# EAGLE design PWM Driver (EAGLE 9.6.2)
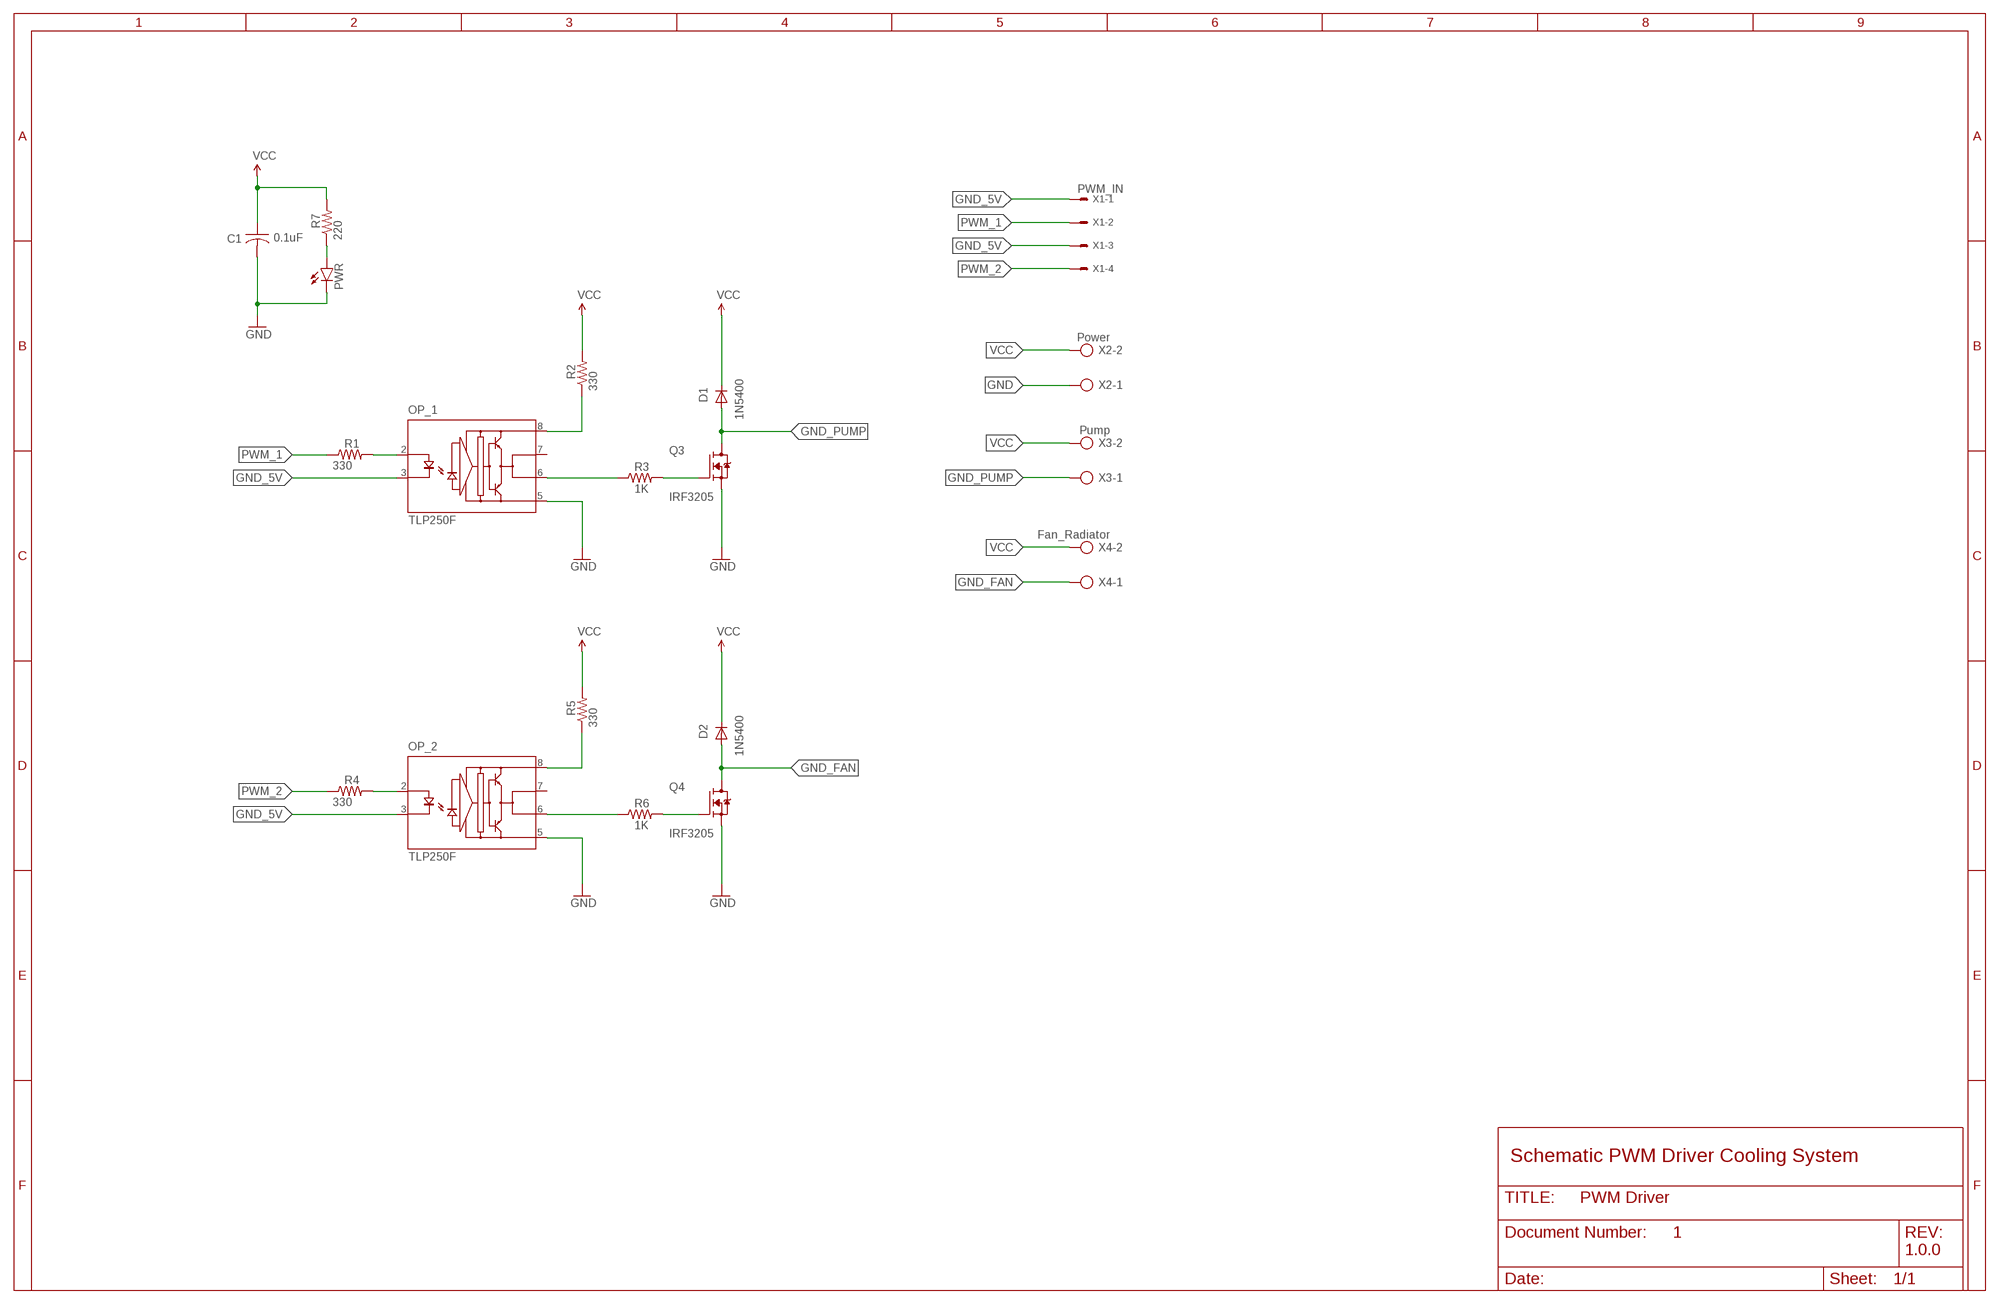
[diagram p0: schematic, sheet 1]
FRAME1 (FRAME_B_L): DESIGNER: PRATIK MAKWANA; DOC: 1; REV: 1.0.0

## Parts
C1  0.1uF  C-US050-030X075  [C050-030X075]
D1  1N5400  [DO201-15]
D2  1N5400  [DO201-15]
OP_1  TLP250F  [DIL08]
OP_2  TLP250F  [DIL08]
PWR  LED5MM  [LED5MM]
Q3  IRF3205  [TO254P1041X444X2933-3]
Q4  IRF3205  [TO254P1041X444X2933-3]
R1  330  R-US_0207/10  [0207/10]
R2  330  R-US_0411/15  [0411/15]
R3  1K  R-US_0411/15  [0411/15]
R4  330  R-US_0207/10  [0207/10]
R5  330  R-US_0411/15  [0411/15]
R6  1K  R-US_0411/15  [0411/15]
R7  220  R-US_0207/10  [0207/10]
X1  PWM_IN  22-23-2041  [22-23-2041]
X2  Power  AK500/2  [AK500/2]
X3  Pump  AK500/2  [AK500/2]
X4  Fan_Radiator  AK500/2  [AK500/2]

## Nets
GND: C1.2 OP_1.5(GND) OP_2.5(GND) PWR.K(C) Q3.3(S) Q4.3(S) X2.1
GND_5V: OP_1.3(K) OP_2.3(K) X1.1 X1.3
GND_FAN: D2.A Q4.2(D) X4.1
GND_PUMP: D1.A Q3.2(D) X3.1
N$1: OP_2.2(A) R4.2
N$2: OP_1.2(A) R1.2
N$3: OP_2.6(VO) R6.1
N$4: OP_1.6(VO) R3.1
N$5: Q3.1(G) R3.2
N$6: PWR.A R7.1
N$7: OP_1.8(VCC) R2.1
N$8: Q4.1(G) R6.2
N$9: OP_2.8(VCC) R5.1
PWM_1: R1.1 X1.2
PWM_2: R4.1 X1.4
VCC: C1.1 D1.C D2.C R2.2 R5.2 R7.2 X2.2 X3.2 X4.2
Unconnected: OP_1.7(VO') OP_2.7(VO')

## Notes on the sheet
- Schematic PWM Driver Cooling System

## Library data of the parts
C1 = adafruit:C-US: CAPACITOR, American symbol
D1 D2 = diode:1N5400: DIODE
OP_1 OP_2 = optocoupler-3-jcn:TLP250F: Toshiba Transistor Inverter Inverter For Air Conditionor IGBT Gate Drive Power MOS FET Gate Drive
PWR = led:LED: LED
Q3 Q4 = IRF3205:IRF3205: N-Channel 55V 75A (Tc) 170W (Tc) Through Hole TO-220AB Check availability; AVAILABILITY: In Stock; CHECK_PRICES: https://www.snapeda.com/parts/IRF3205/Infineon/view-part/?ref=eda; DESCRIPTION: N-Channel 55V 110A (Tc) 200W (Tc) Through Hole TO-220AB; MF: Infineon Technologies; MP: IRF3205; PACKAGE: TO-220 Infineon; PRICE: None; SNAPEDA_LINK: https://www.snapeda.com/parts/IRF3205/Infineon/view-part/?ref=snap
R1-R7 = adafruit:R-US_: RESISTOR, American symbol
X1 = con-molex:22-23-2041: .100" (2.54mm) Center Header - 4 Pin; MF: MOLEX; MPN: 22-23-2041; OC_FARNELL: 1462920; OC_NEWARK: 38C0355
X2-X4 = con-ptr500:AK500/2: CONNECTOR; OC_FARNELL: unknown; OC_NEWARK: unknown

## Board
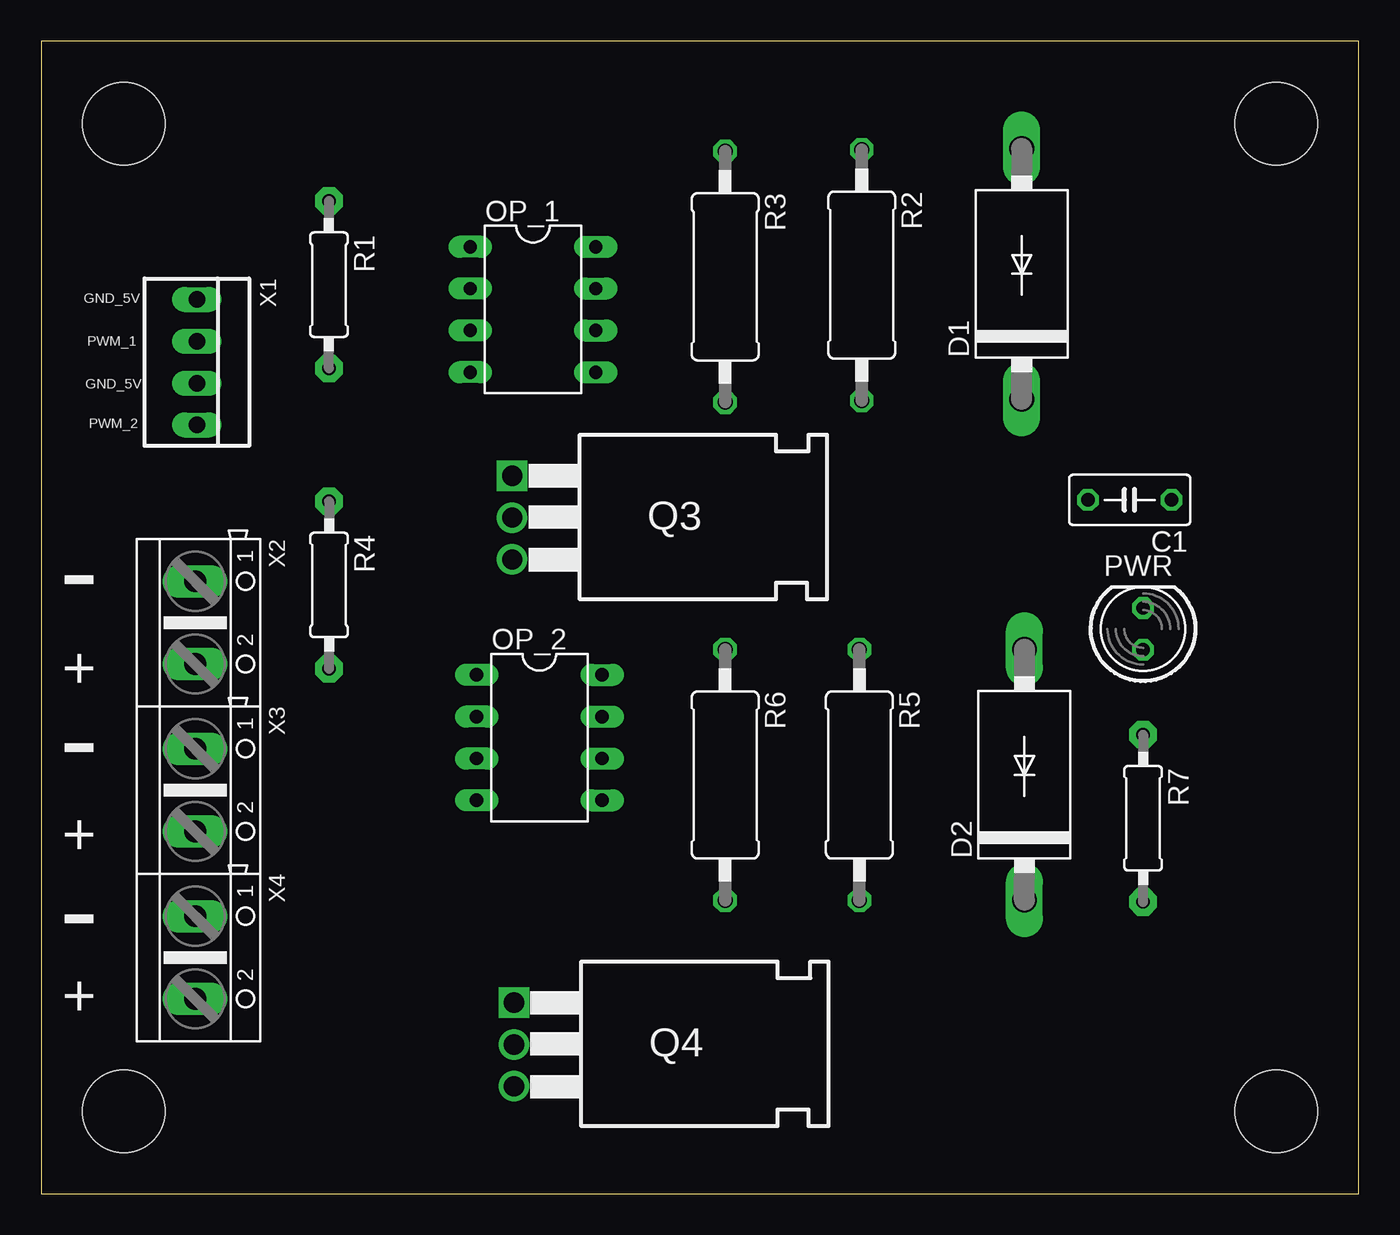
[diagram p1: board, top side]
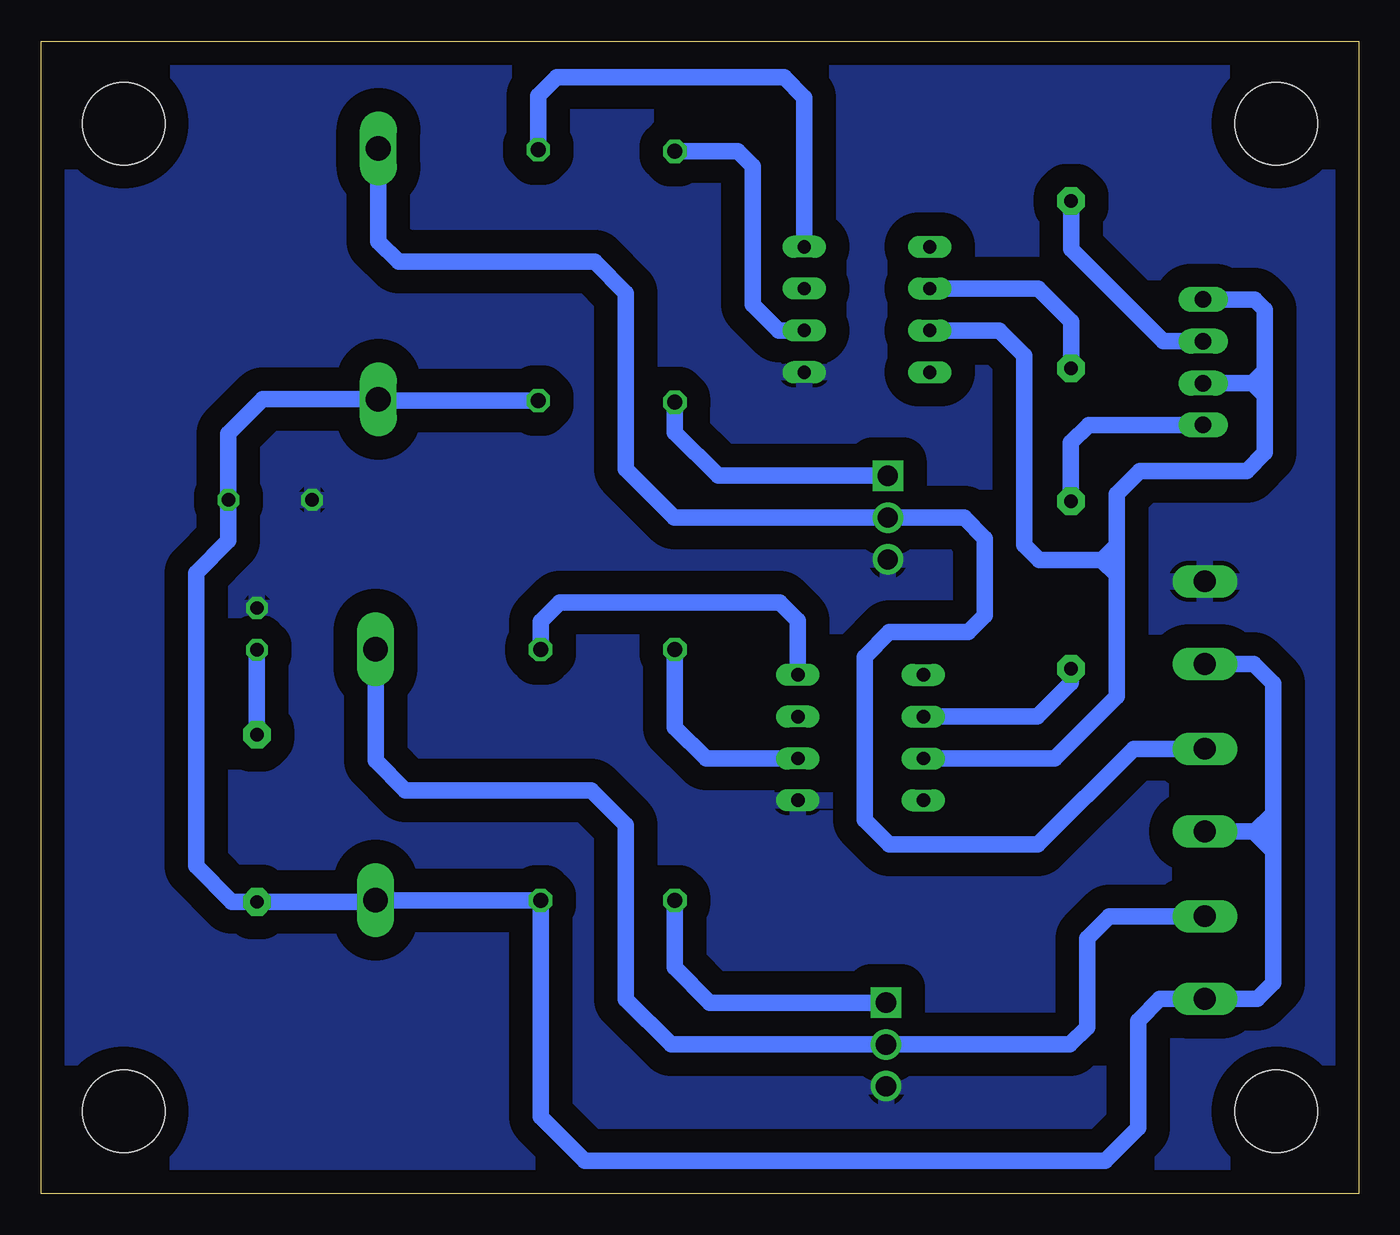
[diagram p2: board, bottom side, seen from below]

Size 80 x 70 mm. Coordinates in mm from the lower left corner, seen from the top.
Outline: 0,0 80,0 80,70 0,70 0,0
Copper layers (1*16): Top 0.035mm / dielectric 1.5mm / Bottom 0.035mm
Design rules "default": minimum track width 6mil, minimum drill 0.35mm, track to track 6mil, track to pad 6mil, pad to pad 6mil, via to via 6mil, smd to smd 6mil, copper to edge 40mil, drill to drill 6mil, minimum pad ring 10mil, minimum via ring 8mil, stop-mask expansion 4mil, vias tented up to drill 0mil, thermal gap 10mil
Holes 5 mm at 5,65 5,5 75,5 75,65

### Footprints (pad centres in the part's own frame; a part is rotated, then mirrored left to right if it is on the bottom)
C050-030X075 = drill 0.813 octagon: 1 -2.54,0; 2 2.54,0
DO201-15 = drill 1.499 long: A 7.62,0; C -7.62,0
DIL08 = drill 0.813 long: 1 -3.81,-3.81; 2 -1.27,-3.81; 3 1.27,-3.81; 4 3.81,-3.81; 5 3.81,3.81; 6 1.27,3.81; 7 -1.27,3.81; 8 -3.81,3.81
LED5MM = drill 0.813 octagon: A -1.27,0; K 1.27,0
TO254P1041X444X2933-3 = drill 1.23 pad 1.85 square: 1 2.5,-4.2 | drill 1.23 pad 1.85: 2 5.04,-4.2; 3 7.58,-4.2
0207/10 = drill 0.813 pad 1.676 octagon: 1 -5.08,0; 2 5.08,0
0411/15 = drill 0.914 octagon: 1 -7.62,0; 2 7.62,0
22-23-2041 = drill 1 long: 1 -3.81,0; 2 -1.27,0; 3 1.27,0; 4 3.81,0
AK500/2 = drill 1.321 long: 1 -2.515,0; 2 2.515,0

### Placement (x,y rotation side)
C1  66.09,42.14 180 top
D1  59.53,55.87 90 top
D2  59.7,25.44 90 top
OP_1  29.86,53.7 270 top
OP_2  30.25,27.7 270 top
PWR  66.9,34.3 90 top
Q3  32.8,46.1 270 top
Q4  32.9,14.1 270 top
R1  17.47,55.21 270 top
R2  49.82,55.79 270 top
R3  41.53,55.69 270 top
R4  17.48,36.97 270 top
R5  49.68,25.43 270 top
R6  41.53,25.43 270 top
R7  66.9,22.8 270 top
X1  9.45,50.5 270 top
X2  9.35,34.68 270 top
X3  9.35,24.51 270 top
X4  9.35,14.34 270 top

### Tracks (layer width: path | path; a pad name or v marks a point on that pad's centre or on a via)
GND
  pour Bottom (isolate 1.422): 0,70 80,70 80,0 0,0
GND_5V
  Bottom 1.016: 14.7,39.4 15.6,38.5 | 15.6,38.5 19.4,38.5 20.3,39.4 20.3,50.9 21.83,52.43 OP_1.3 | OP_2.3 18.47,26.43 14.7,30.2 14.7,37.6 | 14.7,37.6 14.7,39.4 | 15.6,38.5 14.7,37.6 | X1.3 6.47,49.23 | 5.7,50 6.47,49.23 | 5.7,50 5.7,53.7 6.31,54.31 X1.1 | 14.7,39.4 14.7,42.5 13.3,43.9 6.8,43.9 5.7,45 5.7,48.46 | 5.7,48.46 5.7,50 | 6.47,49.23 5.7,48.46
GND_FAN
  Bottom 1.016: D2.A 59.7,26.3 57.9,24.5 46.6,24.5 44.5,22.4 44.5,11.8 41.76,9.06 Q4.2 17.54,9.06 16.5,10.1 16.5,15.5 15.14,16.86 X4.1
GND_PUMP
  Bottom 1.016: X3.1 13.68,27.02 19.5,21.2 28.5,21.2 30,22.7 30,32.6 28.5,34.1 23.7,34.1 22.7,35.1 22.7,39.8 23.96,41.06 Q3.2 41.56,41.06 44.5,44 44.5,54.7 46.4,56.6 58.3,56.6 59.53,57.83 D1.A
N$1
  Bottom 1.016: OP_2.2 19.53,28.97 17.48,31.02 R4.2
N$2
  Bottom 1.016: R1.2 17.47,52.97 19.47,54.97 OP_1.2
N$3
  Bottom 1.016: OP_2.6 39.63,26.43 41.53,28.33 R6.1
N$4
  Bottom 1.016: OP_1.6 35.23,52.43 36.8,54 36.8,62.4 37.71,63.31 R3.1
N$5
  Bottom 1.016: Q3.1 38.9,43.6 41.53,46.23 R3.2
N$6
  Bottom 1.016: PWR.A R7.1
N$7
  Bottom 1.016: R2.1 49.82,66.68 48.7,67.8 34.9,67.8 33.67,66.57 OP_1.8
N$8
  Bottom 1.016: Q4.1 39.4,11.6 41.53,13.73 R6.2
N$9
  Bottom 1.016: OP_2.8 34.06,34.81 35.15,35.9 48.53,35.9 49.68,34.75 R5.1
PWM_1
  Bottom 1.016: R1.1 17.47,57.37 11.87,51.77 X1.2
PWM_2
  Bottom 1.016: R4.1 17.48,45.62 16.41,46.69 X1.4
VCC
  Bottom 1.016: 5.2,20.8 5.2,12.8 6.17,11.82 X4.2 12.07,11.82 13.4,10.5 13.4,4 15.4,2 47,2 49.68,4.68 R5.2 D2.C 59.8,17.72 R7.2 68.42,17.72 70.6,19.9 70.6,37.7 68.63,39.67 C1.1 68.63,46.17 66.55,48.25 D1.C 59.45,48.17 R2.2 | 5.2,20.8 6.39,22 X3.2 6.3,22 5.2,23.1 | X2.2 6.37,32.16 5.2,31 5.2,23.1 | 5.2,23.1 5.2,20.8

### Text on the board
tNames: GND_5V | PWM_1 | GND_5V | PWM_2 | - | + | - | + | - | +

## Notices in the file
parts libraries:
SparkFun: Licensing: CC v3.0 Share-Alike You are welcome to use this library for commercial purposes.
